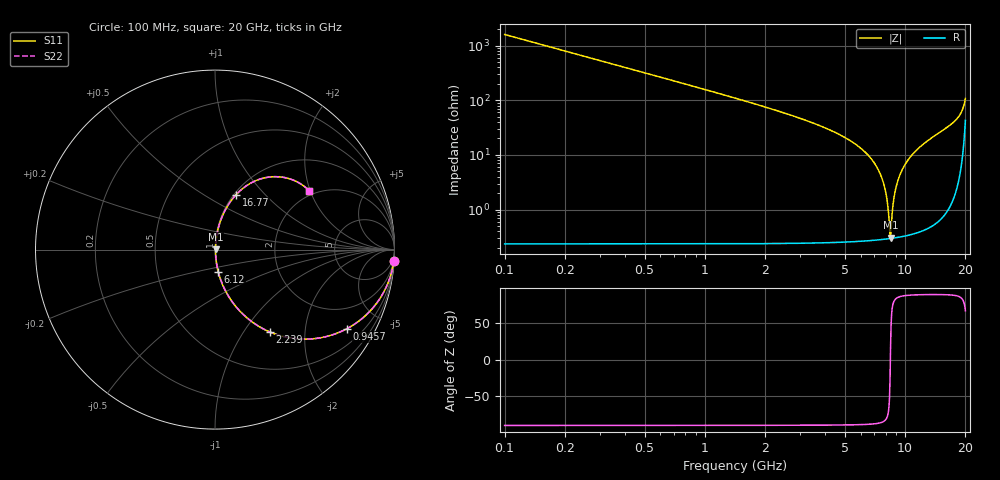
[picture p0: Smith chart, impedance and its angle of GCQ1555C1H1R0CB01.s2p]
!Murata Part Number: GCQ1555C1H1R0CB01
!These Parameters are Measured in Series Mode Connection
!Data Generated on Mar 13, 2026
!  o--ll--o
!Port1  Port2
!  o------o
!Operation Temp=25[degC], DC Bias Voltage=0[V]
!Freq. Start=100[MHz] Stop=20[GHz] 401[Steps]
# Hz S RI R 50
!Freq.(Hz) S11(Real) S11(Imag) S21(Real) S21(Imag) S12(Real) S12(Imag) S22(Real) S22(Imag)
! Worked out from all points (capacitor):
!   401 points, 100 MHz to 20 GHz, reference 50 ohm
!   read as one part in series: C = 1 pF near 199.5 MHz
!   lowest |Z| = 308 mohm at 8.458 GHz (marker M1)
!   series resonance near 8.44 GHz, so ESL is about 360 pH
!   S11 on the Smith chart (normalised r, x): 100 MHz: 1, -32; 945.8 MHz: 1.00, -3.32; 2.239 GHz: 1.00, -1.32; 6.12 GHz: 1.01, -0.25; 16.77 GHz: 1.02, +0.70; 20 GHz: 1.86, +1.97
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1e8  0.9961 -0.0626  0.00394 0.0626  0.00394 0.0626  0.9961 -0.0626
4.4825e8  0.926 -0.2615  0.074 0.2615  0.074 0.2615  0.926 -0.2615
9.4575e8  0.734 -0.4412  0.266 0.4412  0.266 0.4412  0.734 -0.4412
2.23925e9  0.3053 -0.4587  0.6947 0.4587  0.6947 0.4587  0.3053 -0.4587
3.43325e9  0.1327 -0.3361  0.8673 0.3361  0.8673 0.3361  0.1327 -0.3361
6.11975e9  0.0179 -0.1225  0.9821 0.1225  0.9821 0.1225  0.0179 -0.1225
6.7665e9  0.00991 -0.0844  0.9901 0.0844  0.9901 0.0844  0.00991 -0.0844
7.41325e9  0.00528 -0.0497  0.9947 0.0497  0.9947 0.0497  0.00528 -0.0497
7.861e9  0.00361 -0.0273  0.9964 0.0273  0.9964 0.0273  0.00361 -0.0273
8.10975e9  0.00314 -0.0154  0.9969 0.0154  0.9969 0.0154  0.00314 -0.0154
8.3585e9  0.00296 -0.00375  0.997 0.00375  0.997 0.00375  0.00296 -0.00375
8.458e9  0.00296 0.000807  0.997 -0.000807  0.997 -0.000807  0.00296 0.000807
8.7565e9  0.00322 0.0142  0.9968 -0.0142  0.9968 -0.0142  0.00322 0.0142
9.00525e9  0.00369 0.0251  0.9963 -0.0251  0.9963 -0.0251  0.00369 0.0251
9.453e9  0.00511 0.044  0.9949 -0.044  0.9949 -0.044  0.00511 0.044
1.005e10  0.00799 0.0682  0.992 -0.0682  0.992 -0.0682  0.00799 0.0682
1.139325e10  0.0182 0.1191  0.9818 -0.1191  0.9818 -0.1191  0.0182 0.1191
1.338325e10  0.0419 0.1887  0.9581 -0.1887  0.9581 -0.1887  0.0419 0.1887
1.67165e10  0.1157 0.3042  0.8843 -0.3042  0.8843 -0.3042  0.1157 0.3042
1.676625e10  0.1175 0.3061  0.8825 -0.3061  0.8825 -0.3061  0.1175 0.3061
1.8806e10  0.2471 0.3917  0.7529 -0.3917  0.7529 -0.3917  0.2471 0.3917
2e10  0.5257 0.3275  0.4743 -0.3275  0.4743 -0.3275  0.5257 0.3275
